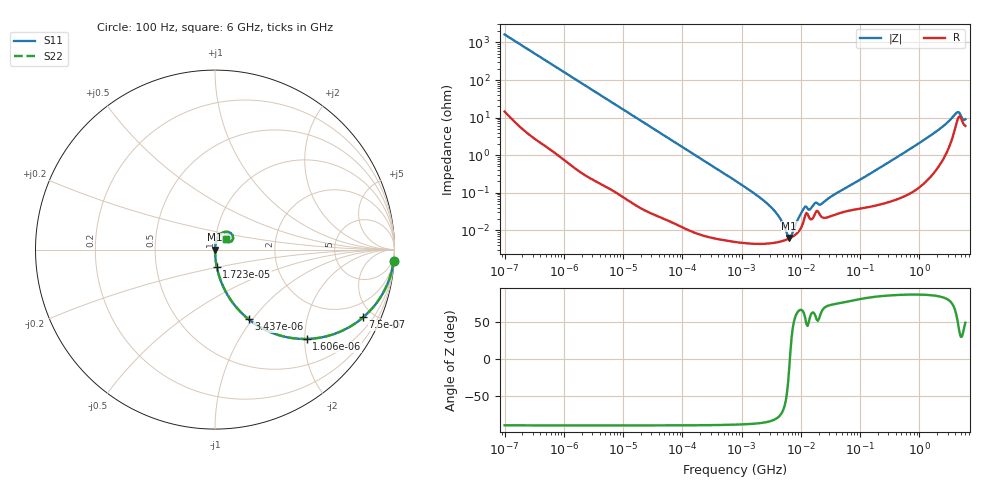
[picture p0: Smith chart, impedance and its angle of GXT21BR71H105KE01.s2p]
!Murata Part Number: GXT21BR71H105KE01
!These Parameters are Measured in Series Mode Connection
!Data Generated on Jan 08, 2026
!  o--ll--o
!Port1  Port2
!  o------o
!Operation Temp=25[degC], DC Bias Voltage=0[V]
!Freq. Start=100[Hz] Stop=6[GHz] 401[Steps]
# Hz S RI R 50
!Freq.(Hz) S11(Real) S11(Imag) S21(Real) S21(Imag) S12(Real) S12(Imag) S22(Real) S22(Imag)
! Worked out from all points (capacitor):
!   401 points, 100 Hz to 6 GHz, reference 50 ohm
!   read as one part in series: C = 977 nF near 109 Hz
!   lowest |Z| = 6.24 mohm at 6.353 MHz (marker M1)
!   series resonance near 6.542 MHz, so ESL is about 610 pH
!   S11 on the Smith chart (normalised r, x): 100 Hz: 1, -33; 750 Hz: 1.02, -4.36; 1.606 kHz: 1.01, -2.04; 3.437 kHz: 1.00, -0.96; 17.23 kHz: 1.00, -0.19; 6 GHz: 1.12, +0.14
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100  0.9957 -0.0612  0.0043 0.0612  0.0043 0.0612  0.9957 -0.0612
350  0.955 -0.2047  0.045 0.2047  0.045 0.2047  0.955 -0.2047
750  0.8251 -0.3774  0.1749 0.3774  0.1749 0.3774  0.8251 -0.3774
1606  0.5103 -0.4978  0.4897 0.4978  0.4897 0.4978  0.5103 -0.4978
2008  0.4004 -0.488  0.5996 0.488  0.5996 0.488  0.4004 -0.488
3437  0.1868 -0.3876  0.8132 0.3876  0.8132 0.3876  0.1868 -0.3876
6728  0.0574 -0.2302  0.9426 0.2302  0.9426 0.2302  0.0574 -0.2302
17227  0.00951 -0.0948  0.9905 0.0948  0.9905 0.0948  0.00951 -0.0948
40335  0.0019 -0.0409  0.9981 0.0409  0.9981 0.0409  0.0019 -0.0409
774597  5.35e-05 -0.00212  0.9999 0.00212  0.9999 0.00212  5.35e-05 -0.00212
2837864  4.47e-05 -0.00048  1 0.00048  1 0.00048  4.47e-05 -0.00048
4060267  4.82e-05 -0.000255  1 0.000255  1 0.000255  4.82e-05 -0.000255
5554849  5.54e-05 -8.56e-05  0.9999 8.56e-05  0.9999 8.56e-05  5.54e-05 -8.56e-05
6353432  6.05e-05 -1.53e-05  0.9999 1.53e-05  0.9999 1.53e-05  6.05e-05 -1.53e-05
7599586  7.1e-05 8.07e-05  0.9999 -8.07e-05  0.9999 -8.07e-05  7.1e-05 8.07e-05
1.137099e7  0.000194 0.000342  0.9998 -0.000342  0.9998 -0.000342  0.000194 0.000342
1.555665e7  0.0002 0.000377  0.9998 -0.000377  0.9998 -0.000377  0.0002 0.000377
2.225763e7  0.00023 0.000448  0.9998 -0.000448  0.9998 -0.000448  0.00023 0.000448
3.124326e8  0.000613 0.00659  0.9994 -0.00659  0.9994 -0.00659  0.000613 0.00659
1.791126e9  0.00496 0.0387  0.995 -0.0387  0.995 -0.0387  0.00496 0.0387
4.193612e9  0.0723 0.0991  0.9277 -0.0991  0.9277 -0.0991  0.0723 0.0991
6e9  0.0605 0.06  0.9395 -0.06  0.9395 -0.06  0.0605 0.06
